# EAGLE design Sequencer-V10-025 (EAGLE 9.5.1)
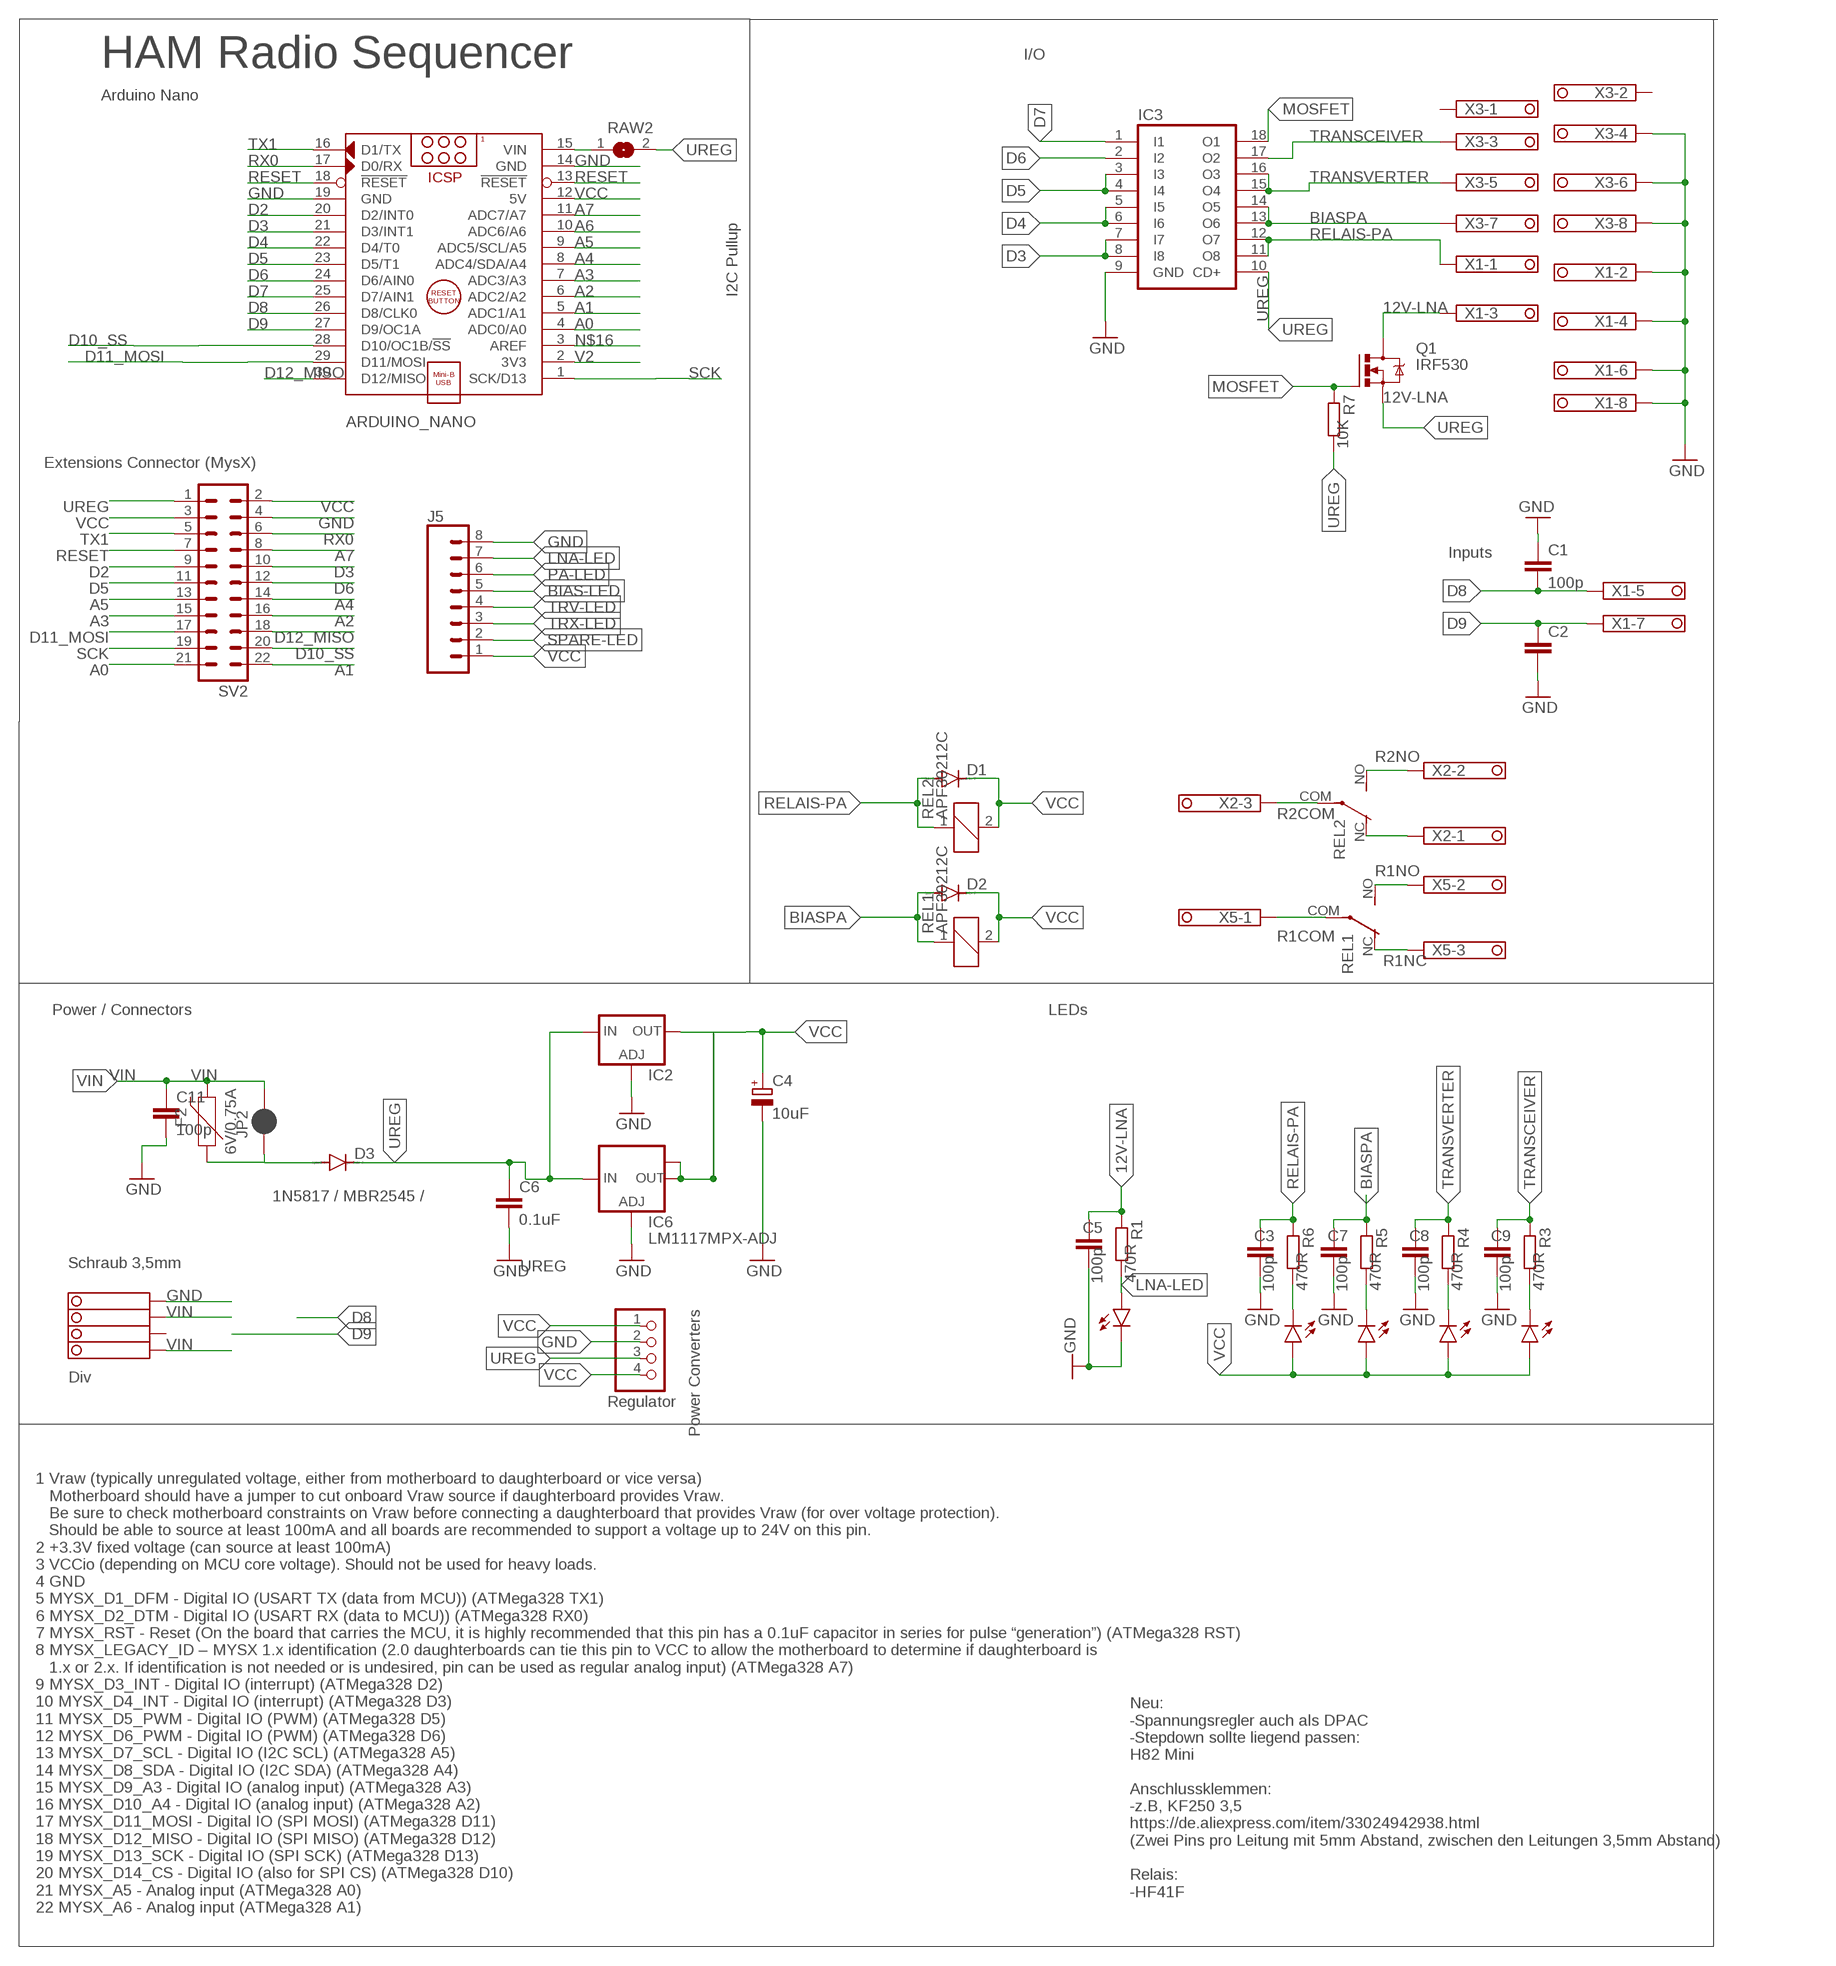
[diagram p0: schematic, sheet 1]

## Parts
ARDUINO_NANO  ARDUINO_NANO_OHNE-BOHR  [ARDUINO_NANO]
C1  100p  C-EU025-025X050  [C025-025X050]
C2  C-EU025-025X050  [C025-025X050]
C3  100p  C-EU025-025X050  [C025-025X050]
C4  10uF  CPOL-EUE3.5-8  [E3,5-8]
C5  100p  C-EU025-025X050  [C025-025X050]
C6  0.1uF  C-EU050-024X044  [C050-024X044]
C7  100p  C-EU025-025X050  [C025-025X050]
C8  100p  C-EU025-025X050  [C025-025X050]
C9  100p  C-EU025-025X050  [C025-025X050]
C11  100p  C-EU025-025X050  [C025-025X050]
D1  DIODE-D-2.5  [D-2.5]
D2  DIODE-D-2.5  [D-2.5]
D3  1N5817 / MBR2545 /  DIODE-D-7.5  [D-7.5]
F2  6V/0.75A  PPTC_THREE-QUARTER-AMP  [1206]
IC2  LD117ADT50TR  [DPACK]
IC3  ULN2803A  [DIL18]
IC6  LM1117MPX-ADJ  [SOT223]
J5  CONN_08LOCK  [1X08_LOCK]
JP2  JUMPER-SMT_2_NC_PASTE_NO-SILK  [SMT-JUMPER_2_NC_PASTE_NO-SILK]
LED-BIAS  LED3MM  [LED3MM]
LED-LNA  LED3MM  [LED3MM]
LED-PA  LED3MM  [LED3MM]
LED-TRV  LED3MM  [LED3MM]
LED-TRX  LED3MM  [LED3MM]
Q1  IRF530  [TO220BV]
R1  470R  R-EU_0207/7  [0207/7]
R3  470R  R-EU_0207/7  [0207/7]
R4  470R  R-EU_0207/7  [0207/7]
R5  470R  R-EU_0207/7  [0207/7]
R6  470R  R-EU_0207/7  [0207/7]
R7  10K  R-EU_0207/7  [0207/7]
RAW2  SJ  [SJ]
REL1  APF30212C  [APF30212C]
REL2  APF30212C  [APF30212C]
STEPDWN  PINHD-1X04_2.54-S  [1X04-S]
SV2  MA11-2  [MA11-2]
X1  MARTIN8X2-1751303  [1751303]
X2  MARTIN3X2-1751303175L303-3  [1751303-3]
X3  MARTIN8X2-1751303  [1751303]
X4  1751264  [1751264]
X5  MARTIN3X2-1751303175L303-3  [1751303-3]

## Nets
12V-LNA: C5.1 Q1.D R1.1 X1.11
A0 [Signal]: ARDUINO_NANO.4(ADC0/A0) SV2.21
A1 [Signal]: ARDUINO_NANO.5(ADC1/A1) SV2.22
A2 [Signal]: ARDUINO_NANO.6(ADC2/A2) SV2.16
A3 [Signal]: ARDUINO_NANO.7(ADC3/A3) SV2.15
A4 [Signal]: ARDUINO_NANO.8(ADC4/SDA/A4) SV2.14
A5 [Signal]: ARDUINO_NANO.9(ADC5/SCL/A5) SV2.13
A6 [Signal]: ARDUINO_NANO.10(ADC6/A6)
A7 [Signal]: ARDUINO_NANO.11(ADC7/A7) SV2.8
BIAS-LED [Signal]: J5.5 LED-BIAS.K(C) R5.2
BIASPA: C7.1 D2.A IC3.13(O6) IC3.14(O5) R5.1 REL1.1 X3.15
D2 [Signal]: ARDUINO_NANO.20(D2/INT0) SV2.9
D3 [Signal]: ARDUINO_NANO.21(D3/INT1) IC3.7(I7) IC3.8(I8) SV2.10
D4 [Signal]: ARDUINO_NANO.22(D4/T0) IC3.5(I5) IC3.6(I6)
D5 [Signal]: ARDUINO_NANO.23(D5/T1) IC3.3(I3) IC3.4(I4) SV2.11
D6 [Signal]: ARDUINO_NANO.24(D6/AIN0) IC3.2(I2) SV2.12
D7 [Signal]: ARDUINO_NANO.25(D7/AIN1) IC3.1(I1)
D8 [Signal]: ARDUINO_NANO.26(D8/CLK0) C1.2 X1.13
D9 [Signal]: ARDUINO_NANO.27(D9/OC1A) C2.1 X1.15
D10_SS [Signal]: ARDUINO_NANO.28(D10/OC1B/!SS) SV2.20
D11_MOSI [Signal]: ARDUINO_NANO.29(D11/MOSI) SV2.17
D12_MISO [Signal]: ARDUINO_NANO.30(D12/MISO) SV2.18
GND [Power]: ARDUINO_NANO.14(GND) ARDUINO_NANO.19(GND) C1.1 C2.2 C3.2 C4.- C5.2 C6.2 C7.2 C8.2 C9.2 C11.2 IC2.1(ADJ) IC3.9(GND) IC6.1(ADJ) J5.8 LED-LNA.K(C) STEPDWN.2 SV2.4 X1.10 X1.12 X1.14 X1.16 X3.12 X3.14 X3.16 X4.4
LNA-LED [Signal]: J5.7 LED-LNA.A R1.2
MOSFET: IC3.18(O1) Q1.G R7.1
N$1: D3.A F2.1 JP2.1
N$16: ARDUINO_NANO.3(AREF)
PA-LED [Signal]: J5.6 LED-PA.K(C) R6.2
R1COM: REL1.COM(2:P) X5.1
R1NC: REL1.NC(2:O) X5.3
R1NO: REL1.NO(2:S) X5.2
R2COM: REL2.COM(2:P) X2.3
R2NC: REL2.NC(2:O) X2.1
R2NO: REL2.NO(2:S) X2.2
RAW1 [Power]: ARDUINO_NANO.15(VIN) RAW2.1
RELAIS-PA: C3.1 D1.A IC3.11(O8) IC3.12(O7) R6.1 REL2.1 X1.9
RESET [Signal]: ARDUINO_NANO.13(!RESET) ARDUINO_NANO.18(!RESET) SV2.7
RX0 [Signal]: ARDUINO_NANO.17(D0/RX) SV2.6
SCK [Signal]: ARDUINO_NANO.1(SCK/D13) SV2.19
SPARE-LED [Signal]: J5.2
TRANSCEIVER: C9.1 IC3.17(O2) R3.1 X3.11
TRANSVERTER: C8.1 IC3.15(O4) IC3.16(O3) R4.1 X3.13
TRV-LED [Signal]: J5.4 LED-TRV.K(C) R4.2
TRX-LED [Signal]: J5.3 LED-TRX.K(C) R3.2
TX1 [Signal]: ARDUINO_NANO.16(D1/TX) SV2.5
UREG [Power]: C6.1 D3.C IC2.3(IN) IC3.10(CD+) IC6.3(IN) Q1.S R7.2 RAW2.2 STEPDWN.3 SV2.1
V2 [Power]: ARDUINO_NANO.2(3V3)
VCC [Power]: ARDUINO_NANO.12(5V) C4.+ D1.C D2.C IC2.4(OUT) IC6.2(OUT) IC6.TAB(OUT1) J5.1 LED-BIAS.A LED-PA.A LED-TRV.A LED-TRX.A REL1.2 REL2.2 STEPDWN.1 STEPDWN.4 SV2.2 SV2.3
VIN [Power]: C11.1 F2.2 JP2.2 X4.1 X4.3
Unconnected: X3.9 X3.10 X4.2

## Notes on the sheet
- I/O
- HAM Radio Sequencer
- Arduino Nano
- I2C Pullup
- Extensions Connector (MysX)
- Inputs
- Power / Connectors | LEDs
- Schraub 3,5mm
- Power Converters
- Div
- Regulator
- Neu:
  -Spannungsregler auch als DPAC
  -Stepdown sollte liegend passen:  
  H82 Mini
  
  Anschlussklemmen:
  -z.B, KF250 3,5 
  https://de.aliexpress.com/item/33024942938.html
  (Zwei Pins pro Leitung mit 5mm Abstand, zwischen den Leitungen 3,5mm Abstand)
  
  Relais:
  -HF41F
- 1 Vraw (typically unregulated voltage, either from motherboard to daughterboard or vice versa)
     Motherboard should have a jumper to cut onboard Vraw source if daughterboard provides Vraw. 
     Be sure to check motherboard constraints on Vraw before connecting a daughterboard that provides Vraw (for over voltage protection). 
     Should be able to source at least 100mA and all boards are recommended to support a voltage up to 24V on this pin.
  2 +3.3V fixed voltage (can source at least 100mA)
  3 VCCio (depending on MCU core voltage). Should not be used for heavy loads.
  4 GND
  5 MYSX_D1_DFM - Digital IO (USART TX (data from MCU)) (ATMega328 TX1)
  6 MYSX_D2_DTM - Digital IO (USART RX (data to MCU)) (ATMega328 RX0)
  7 MYSX_RST - Reset (On the board that carries the MCU, it is highly recommended that this pin has a 0.1uF capacitor in series for pulse “generation”) (ATMega328 RST)
  8 MYSX_LEGACY_ID – MYSX 1.x identification (2.0 daughterboards can tie this pin to VCC to allow the motherboard to determine if daughterboard is 
     1.x or 2.x. If identification is not needed or is undesired, pin can be used as regular analog input) (ATMega328 A7)
  9 MYSX_D3_INT - Digital IO (interrupt) (ATMega328 D2)
  10 MYSX_D4_INT - Digital IO (interrupt) (ATMega328 D3)
  11 MYSX_D5_PWM - Digital IO (PWM) (ATMega328 D5)
  12 MYSX_D6_PWM - Digital IO (PWM) (ATMega328 D6)
  13 MYSX_D7_SCL - Digital IO (I2C SCL) (ATMega328 A5)
  14 MYSX_D8_SDA - Digital IO (I2C SDA) (ATMega328 A4)
  15 MYSX_D9_A3 - Digital IO (analog input) (ATMega328 A3)
  16 MYSX_D10_A4 - Digital IO (analog input) (ATMega328 A2)
  17 MYSX_D11_MOSI - Digital IO (SPI MOSI) (ATMega328 D11)
  18 MYSX_D12_MISO - Digital IO (SPI MISO) (ATMega328 D12)
  19 MYSX_D13_SCK - Digital IO (SPI SCK) (ATMega328 D13)
  20 MYSX_D14_CS - Digital IO (also for SPI CS) (ATMega328 D10)
  21 MYSX_A5 - Analog input (ATMega328 A0)
  22 MYSX_A6 - Analog input (ATMega328 A1)

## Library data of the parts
ARDUINO_NANO = ArduinoNanoV30:ARDUINO_NANO_OHNE-BOHR: Arduino Nano V3.0 Module Overview: The Arduino Nano is a small, complete, and breadboard-friendly board based on the ATmega328 (Arduino Nano 3.x) or ATmega168 (Arduino Nano 2.x). It has more or less the same functionality of the Arduino Duemilanove, but in a different package. It lacks only a DC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
C1-C3 C5-C9 C11 = rcl:C-EU: CAPACITOR, European symbol; SPICEPREFIX: C
C4 = rcl:CPOL-EU: POLARIZED CAPACITOR, European symbol; SPICEPREFIX: C
D1-D3 = diode:DIODE-: DIODE
F2 = SparkFun-Fuses:PPTC: Resettable Fuse PPTC; PROD_ID: RES-11150
IC2 = v-reg:LD117A?*: Low drop fixed and adjustable positive voltage regulators 1 A Source: http://www.st.com/stonline/products/literature/ds/7194/ld1117axx.pdf
IC3 = uln-udn:ULN2803A: DRIVER ARRAY
IC6 = lm1117:LM1117MPX-ADJ
J5 = SparkFun-Connectors:CONN_08: Multi connection point. Often used as Generic Header-pin footprint for 0.1 inch spaced/style header connections On any of the 0.1 inch spaced packages, you can populate with these: Break Away Headers - Straight (PRT-00116) Break Away Male Headers - Right Angle (PRT-00553) Female Headers (PRT-00115)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
JP2 = SparkFun-Jumpers:JUMPER-SMT_2_NC_PASTE: Normally closed solder jumper
LED-BIAS LED-LNA LED-PA LED-TRV LED-TRX = led:LED: LED
Q1 = transistor-power:IRF530: HEXFET Power MOSFET
R1 R3-R7 = rcl:R-EU_: RESISTOR, European symbol; SPICEPREFIX: R
RAW2 = jumper:SJ: SMD solder JUMPER
REL1 REL2 = relay:APF30212C: Compliant with European standards 1a/1c 6A Slim power relays Source: Data sheet; OC_FARNELL: unknown
STEPDWN = pinhead-2:PINHD-1X04: PIN HEADER
SV2 = con-Pinheader:MA11-2: PIN HEADER; OC_FARNELL: unknown; OC_NEWARK: unknown
X1 X3 = con-phoenix-350-Martin:MARTIN8X2-1751303: MKDS 1/ 8-3,5 Printklemme Nennstrom: 10 A Bemessungsspannung: 160 V Raster: 3,5 mm Polzahl: 8 Montageart: Löten Anschlussart: Schraubanschluss Anschlussrichtung vom Leiter zur Platine: 0° Source: http://eshop.phoenixcontact.com .. .pdf; OC_FARNELL: unknown; OC_NEWARK: unknown
X2 X5 = con-phoenix-350-Martin:MARTIN3X2-1751303: MKDS 1/ 8-3,5 Printklemme Nennstrom: 10 A Bemessungsspannung: 160 V Raster: 3,5 mm Polzahl: 8 Montageart: Löten Anschlussart: Schraubanschluss Anschlussrichtung vom Leiter zur Platine: 0° Source: http://eshop.phoenixcontact.com .. .pdf
X4 = con-phoenix-350:1751264: MKDS 1/ 4-3,5 Printklemme Nennstrom: 10 A Bemessungsspannung: 160 V Raster: 3,5 mm Polzahl: 4 Montageart: Löten Anschlussart: Schraubanschluss Anschlussrichtung vom Leiter zur Platine: 0° Source: http://eshop.phoenixcontact.com .. 1751264.pdf; MPN: 1751264; OC_FARNELL: unknown; OC_NEWARK: 10R0934

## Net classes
0 default: width 1.219 mm
1 Power: width 0.762 mm
2 Signal: width 0.305 mm

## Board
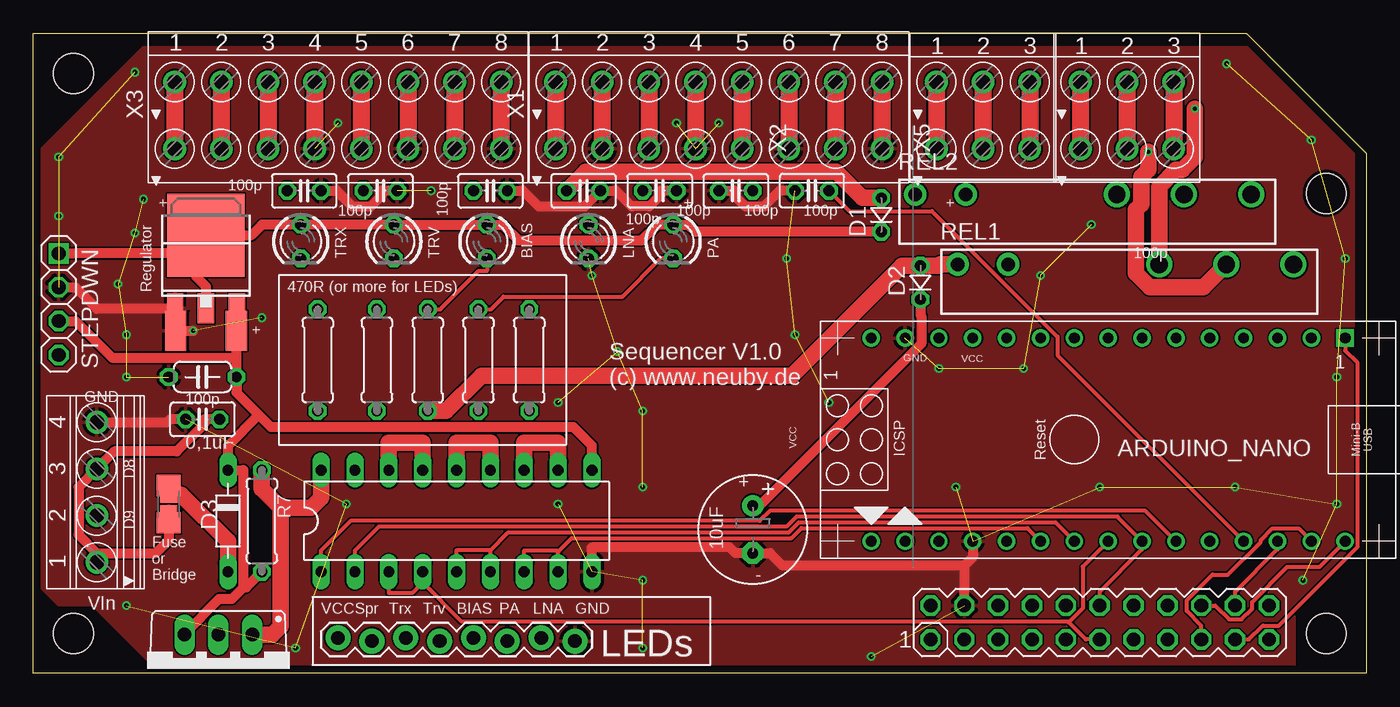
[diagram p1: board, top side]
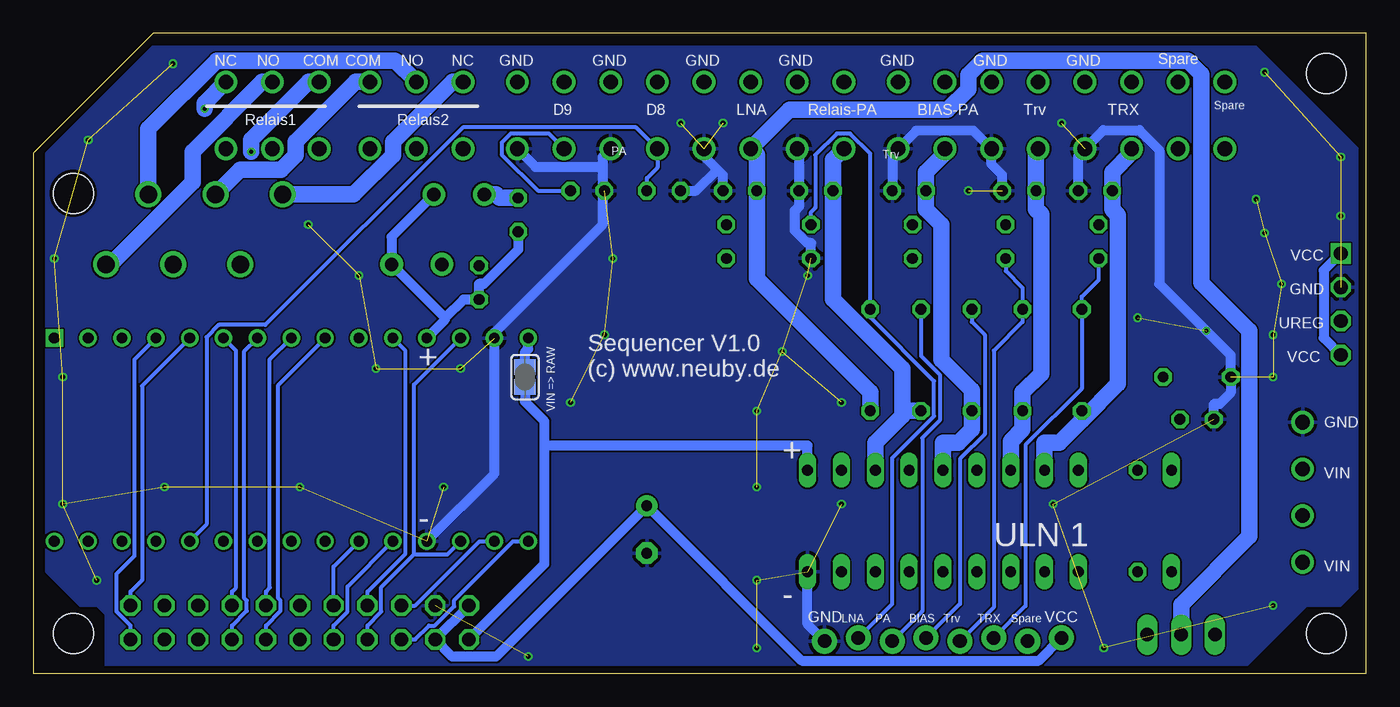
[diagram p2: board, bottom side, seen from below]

Size 100 x 48 mm. Coordinates in mm from the lower left corner, seen from the top.
Outline: 100,0 0,0 0,48 91,48 100,39 100,0
Copper layers (1*16): Top 0.035mm / dielectric 1.5mm / Bottom 0.035mm
Design rules "dirt_cheap_dirty_boards.v1": minimum track width 5mil, minimum drill 12mil, track to track 5mil, track to pad 5mil, pad to pad 5mil, via to via 5mil, smd to smd 0mil, copper to edge 10mil, drill to drill 10mil, minimum pad ring 10mil, minimum via ring 6mil, stop-mask expansion 2mil, vias tented up to drill 25mil, thermal gap 10mil
Holes 3 mm at 3,45 97,36 97,3 3,3

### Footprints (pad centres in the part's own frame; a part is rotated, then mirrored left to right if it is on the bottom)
ARDUINO_NANO = drill 0.8 square: 1 -20.32,-7.62 | drill 0.8: 2 -17.78,-7.62; 3 -15.24,-7.62; 4 -12.7,-7.62; 5 -10.16,-7.62; 6 -7.62,-7.62; 7 -5.08,-7.62; 8 -2.54,-7.62; 9 0,-7.62; 10 2.54,-7.62; 11 5.08,-7.62; 12 7.62,-7.62; 13 10.16,-7.62; 14 12.7,-7.62; 15 15.24,-7.62; 16 15.24,7.62; 17 12.7,7.62; 18 10.16,7.62; 19 7.62,7.62; 20 5.08,7.62; 21 2.54,7.62; 22 0,7.62; 23 -2.54,7.62; 24 -5.08,7.62; 25 -7.62,7.62; 26 -10.16,7.62; 27 -12.7,7.62; 28 -15.24,7.62; 29 -17.78,7.62; 30 -20.32,7.62
C025-025X050 = drill 0.813 octagon: 1 -1.27,0; 2 1.27,0
E3,5-8 = drill 0.813 pad 1.6: + -1.778,0 | drill 0.813 pad 1.6 octagon: - 1.778,0
C050-024X044 = drill 0.813 octagon: 1 -2.54,0; 2 2.54,0
D-2.5 = drill 0.813 octagon: A 1.27,0; C -1.27,0
D-7.5 = drill 0.813 long: A 3.81,0; C -3.81,0
1206 = smd 1.6 x 1.8: 1 -1.4,0; 2 1.4,0
DPACK = smd 1.6 x 3: 1 -2.28,-4.8; 3 2.28,-4.8 | smd 5.8 x 6.2: 4 0,2.38
DIL18 = drill 0.813 long: 1 -10.16,-3.81; 2 -7.62,-3.81; 3 -5.08,-3.81; 4 -2.54,-3.81; 5 0,-3.81; 6 2.54,-3.81; 7 5.08,-3.81; 8 7.62,-3.81; 9 10.16,-3.81; 10 10.16,3.81; 11 7.62,3.81; 12 5.08,3.81; 13 2.54,3.81; 14 0,3.81; 15 -2.54,3.81; 16 -5.08,3.81; 17 -7.62,3.81; 18 -10.16,3.81
SOT223 = smd 1.219 x 2.235: 1 -2.311,-3.099; 2 0,-3.099; 3 2.311,-3.099 | smd 3.6 x 2.2: TAB 0,3.099
1X08_LOCK = drill 1.016 pad 1.88: 1 0,0.127; 2 2.54,-0.127; 3 5.08,0.127; 4 7.62,-0.127; 5 10.16,0.127; 6 12.7,-0.127; 7 15.24,0.127; 8 17.78,-0.127
SMT-JUMPER_2_NC_PASTE_NO-SILK = smd 0.635 x 1.27: 1 -0.406,0; 2 0.406,0
LED3MM = drill 0.813 octagon: A -1.27,0; K 1.27,0
TO220BV = drill 1.016 long: D 0,-2.54; G -2.54,-2.54; S 2.54,-2.54
0207/7 = drill 0.813 octagon: 1 -3.81,0; 2 3.81,0
SJ = smd 1.168 x 1.6: 1 -0.762,0; 2 0.762,0
APF30212C = drill 1 pad 1.7: 1 -12.6,0; 2 -8.82,0 | drill 1.3 pad 1.9: COM 7.56,0; NC 2.52,0; NO 12.6,0
1X04-S = drill 1.016 square: 1 -3.81,0 | drill 1.016 octagon: 2 -1.27,0; 3 1.27,0; 4 3.81,0
MA11-2 = drill 1.016 octagon: 1 -12.7,-1.27; 2 -12.7,1.27; 3 -10.16,-1.27; 4 -10.16,1.27; 5 -7.62,-1.27; 6 -7.62,1.27; 7 -5.08,-1.27; 8 -5.08,1.27; 9 -2.54,-1.27; 10 -2.54,1.27; 11 0,-1.27; 12 0,1.27; 13 2.54,-1.27; 14 2.54,1.27; 15 5.08,-1.27; 16 5.08,1.27; 17 7.62,-1.27; 18 7.62,1.27; 19 10.16,-1.27; 20 10.16,1.27; 21 12.7,-1.27; 22 12.7,1.27
1751303 = drill 1.1 pad 1.7: 1 -12.25,-0.1; 2 -8.75,-0.1; 3 -5.25,-0.1; 4 -1.75,-0.1; 5 1.75,-0.1; 6 5.25,-0.1; 7 8.75,-0.1; 8 12.25,-0.1; 9 -12.25,-5.1; 10 -8.75,-5.1; 11 -5.25,-5.1; 12 -1.75,-5.1; 13 1.75,-5.1; 14 5.25,-5.1; 15 8.75,-5.1; 16 12.25,-5.1
1751303-3 = drill 1.1 pad 1.7: 1 -3.36,2.44; 2 0.14,2.44; 3 3.64,2.44; 4 -3.36,-2.56; 5 0.14,-2.56; 6 3.64,-2.56
1751264 = drill 1.1 pad 1.7: 1 -5.25,-0.1; 2 -1.75,-0.1; 3 1.75,-0.1; 4 5.25,-0.1

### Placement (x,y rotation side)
ARDUINO_NANO  78.11,17.52 180 top
C1  52.7,36.2 0 top
C2  58.42,36.2 180 top
C3  41.27,36.2 0 top
C4  53.98,10.79 270 top
C5  46.99,36.2 0 top
C6  12.7,22.23 180 top
C7  34.29,36.2 0 top
C8  26.04,36.2 0 top
C9  20.32,36.2 0 top
C11  12.7,19.05 180 top
D1  63.62,34.38 90 top
D2  66.56,29.3 90 top
D3  14.61,11.43 270 top
F2  10.16,12.7 270 top
IC2  12.96,30.48 0 top
IC3  31.75,11.43 0 top
IC6  12.96,30.48 0 top
J5  22.86,2.54 0 top
JP2  10.16,12.7 270 top
LED-BIAS  34.03,32.38 270 top
LED-LNA  41.66,32.38 270 top
LED-PA  48.01,32.38 270 top
LED-TRV  27.05,32.38 270 top
LED-TRX  20.07,32.38 270 top
Q1  13.88,0.36 180 top
R1  37.21,23.5 90 top
R3  21.34,23.5 90 top
R4  25.78,23.5 90 top
R5  29.59,23.5 90 top
R6  33.4,23.5 90 top
R7  17.14,11.43 270 top
RAW2  63.12,22.23 270 bottom
REL1  81.94,30.68 0 top
REL2  78.77,35.91 0 top
STEPDWN  1.91,27.68 270 top
SV2  80.01,3.81 0 top
X1  51.44,44.45 0 top
X2  71.12,41.91 0 top
X3  22.86,44.45 0 top
X4  4.67,13.59 90 top
X5  81.92,41.91 0 top

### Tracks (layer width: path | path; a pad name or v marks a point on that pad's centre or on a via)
12V-LNA
  Bottom 1.219: Q1.D 13.88,5.16 8.76,10.29 8.76,25.68 12.36,29.28 12.36,44.93 13.38,45.95 28.79,45.95 29.86,44.88 29.86,43.81 31.41,42.26 43.27,42.26 X1.11 45.72,38.88 C5.1 45.72,29.59 37.21,21.08 R1.1
A0
  Bottom 0.305: SV2.21 92.71,3.58 93.75,4.62 93.75,7.47 92.41,8.81 92.41,23.54 ARDUINO_NANO.4
A1
  Bottom 0.305: ARDUINO_NANO.5 91.85,21.56 91.85,6.99 92.71,6.12 SV2.22
A2
  Bottom 0.305: SV2.16 85.09,6.12 84.78,6.43 84.78,24.2 ARDUINO_NANO.6
A3
  Bottom 0.305: SV2.15 85.09,3.58 83.99,4.68 83.99,5.46 84.17,5.63 84.17,24.16 ARDUINO_NANO.7
A4
  Bottom 0.305: SV2.14 82.55,6.12 82.25,6.42 82.25,23.54 ARDUINO_NANO.8
A5
  Bottom 0.305: SV2.13 82.55,3.58 81.45,4.68 81.45,5.46 81.63,5.63 81.63,21.62 ARDUINO_NANO.9
A7
  Bottom 0.305: SV2.8 74.93,6.12 72.07,8.98 72.07,24.19 ARDUINO_NANO.11
BIAS-LED
  Top 0.305: LED-BIAS.K 34.03,30.18 33.4,30.18 30.53,27.3 R5.2
  Bottom 0.305: R5.2 29.59,26.36 28.62,25.39 28.62,17.94 30.48,16.08 30.48,5.21 J5.5
BIASPA
  Top 1.219: IC3.13 34.29,17.3 31.75,17.3 IC3.14 | R5.1 30.99,19.68 33.62,22.32 56.91,22.32 65.16,30.57 D2.A 67.26,30.57 67.96,30.57 68.06,30.68 REL1.1
  Bottom 1.219: IC3.14 31.75,17.3 30.58,17.3 29.59,18.29 R5.1 29.59,21.25 31.88,23.54 31.88,33.66 33.02,34.8 C7.1 33.02,37.59 31.61,39 X3.15
D2
  Bottom 0.305: SV2.9 77.47,3.58 76.43,4.62 76.43,6.5 ARDUINO_NANO.20
D3
  Top 0.305: 39.37,9.11 40.39,10.13 56.86,10.13 57.62,10.89 74.58,10.89 ARDUINO_NANO.21 | 39.37,9.11 39.26,9.22 36.83,9.22 IC3.7 | IC3.8 39.37,9.11
  Bottom 0.305: SV2.10 77.47,8 ARDUINO_NANO.21
D4
  Top 0.305: 34.29,9.22 35.64,10.57 56.69,10.57 57.44,11.32 76.69,11.32 ARDUINO_NANO.22 | 34.29,9.22 | IC3.6 34.29,9.11 34.29,9.22 | IC3.5 31.75,9.22 34.29,9.22
D5
  Top 0.305: 77.69,3.82 77.62,3.89 32.14,3.89 29.21,6.82 | 77.69,3.82 78.97,2.54 SV2.11 | ARDUINO_NANO.23 78.74,8 78.74,4.87 77.69,3.82 | IC3.3 26.67,6.02 28.41,6.02 29.21,6.82 | IC3.4 29.21,6.82
D6
  Top 0.305: IC3.2 24.13,9.22 25.91,11 56.51,11 57.26,11.76 81.33,11.76 ARDUINO_NANO.24 83.19,9.3 80.01,6.12 SV2.12
D7
  Top 0.305: ARDUINO_NANO.25 83.44,12.19 55.25,12.19 54.49,11.43 23.8,11.43 21.59,9.22 IC3.1
D8
  Bottom 0.305: ARDUINO_NANO.26 87,11.18 87,25.23 86.09,26.13 82.59,26.13 67.77,40.95 54.79,40.95 X1.13 53.19,37.92 53.98,37.13 53.98,36.66 C1.2
D9
  Top 0.305: C2.1 61.23,34.66 67.43,34.66 76.83,25.26 76.83,23.88 ARDUINO_NANO.27
  Bottom 0.305: X1.15 61.31,40.48 64.17,40.48 64.86,39.8 64.86,38.9 62.15,36.2 C2.1
D10_SS
  Top 0.305: SV2.20 90.17,6.12 93.34,9.3 ARDUINO_NANO.28
D11_MOSI
  Top 0.305: SV2.17 87.63,3.58 86.53,4.68 86.53,5.47 88.46,7.39 89.62,7.39 92.08,9.85 92.08,9.97 92.97,10.86 94.93,10.86 ARDUINO_NANO.29
D12_MISO
  Top 0.305: SV2.18 88.67,5.08 89.71,4.04 90.64,4.04 91.44,4.83 91.44,5.34 94.08,7.98 96.5,7.98 ARDUINO_NANO.30
GND  (via drill 0.3 pad 0.61, 0.35)  (41 unrouted)
  Top 0.762: C11.2 10.26,19.05 10.05,18.84 X4.4 | STEPDWN.2 3.17,28.95 4.79,27.34 10.64,27.34 | 10.64,27.34 10.64,27.3 10.64,27.12 10.64,25.75 10.68,25.72 IC2.1 v11.98,25.68 | IC6.1 10.64,27.34 | C7.2 36.73,36.2 37.91,35.01 41.36,35.01 C3.2 43.71,36.2 44.88,35.03 46.22,35.03 47.09,35.9 47.09,36.2 C5.2 | 69.85,8.09 56.21,8.09 55.28,9.02 C4.- 52.67,9.02 52.23,9.45 41.91,9.45 IC3.9 | ARDUINO_NANO.19 70.48,8.72 69.85,8.09 | 69.85,8.09 69.85,6.35 SV2.4 | C8.2 26.14,36.2 26.14,35.83 25.33,35.03 23.93,35.03 22.76,36.2 C9.2 | C1.1 52.6,36.2 52.6,35.83 53.44,34.99 54.78,34.99 55.98,36.2 C2.2
  Bottom 0.762: 57.26,36.2 57.26,33.7 65.41,25.55 ARDUINO_NANO.14 65.41,14.98 ARDUINO_NANO.19 | 57.26,37.99 57.26,38.77 X1.14 | 57.26,36.2 57.26,37.99 | X1.16 62.32,37.99 57.26,37.99 | C2.2 57.26,36.2 | C11.2 11.43,20.22 11,20.22 10.16,21.06 C6.2 10.16,23.86 v11.98,25.68 15.52,29.22 15.52,39.24 17.02,40.73 19.73,40.73 X3.12 21.59,38.87 C9.2 | 48.68,37.78 48.26,37.36 C5.2 | X1.12 49.69,38.79 48.68,37.78 | 48.68,37.78 50.27,36.2 C1.1 | C8.2 27.3,37.36 28.11,38.17 X3.14 29.47,40.71 33.75,40.71 X3.16 35.56,38.9 C7.2 | LED-LNA.K 41.66,32.28 41.95,32.28 42.86,33.2 42.86,34.71 42.55,35.03 C3.2 42.55,39.21 X1.10 | J5.8 41.91,3.68 IC3.9
  other vias: 1.91,38.73 7.62,45.09 7.62,33.02 6.35,29.21 6.99,25.4 6.99,22.23 6.99,5.08 19.68,1.91 23.5,12.7 17.14,26.67 29.84,36.2 41.91,29.84 43.81,24.13 39.37,20.32 59.69,20.32 39.37,12.7 45.72,1.91 45.72,6.99 45.72,13.97 45.72,19.68 56.52,31.11 57.15,25.4 62.87,1.27 69.22,13.97 67.94,22.86 75.56,29.84 79.38,33.66 89.53,45.72 95.89,40.01 98.42,31.11 97.79,22.23 97.79,12.7 90.17,13.97 80.01,13.97 74.3,22.86 95.25,6.99 1.91,34.29 8.26,35.56 22.86,41.27 48.26,41.27 51.44,41.27
  pour Top: 0.64,6.35 0.64,39.37 8.26,46.99 91.08,46.99 99.06,39.01 99.06,7.62 96.52,5.08 95.25,5.08 94.61,4.45 94.61,0.64 8.89,0.64 4.45,5.08 1.91,5.08
  pour Bottom: 8.89,0.64 4.45,5.08 1.91,5.08 0.64,6.35 0.64,39.37 8.26,46.99 91.08,46.99 99.06,39.01 99.06,7.62 96.52,5.08 95.25,5.08 94.61,4.45 94.61,0.64
LNA-LED
  Bottom 0.305: J5.7 35.56,5.21 35.56,16.15 32.43,19.29 32.43,21.91 37.21,26.69 R1.2 37.21,38.97 38.72,40.48 39.72,40.48 41.32,38.88 41.32,34.93 41.66,34.59 LED-LNA.A
MOSFET
  Top 1.219: 18.56,12.43 17.14,13.84 R7.1 | 18.56,12.43 18.56,3.54 17.92,2.9 Q1.G | 18.56,12.43 20.84,12.43 21.59,13.18 IC3.18
N$1
  Top 0.635: 10.16,13.4 JP2.1
  Top 1.219: D3.A 14.61,9.89 11.1,13.4 10.16,13.4 F2.1
PA-LED
  Top 0.305: LED-PA.K 47.06,31.11 44.2,28.25 35.28,28.25 34.34,27.3 R6.2
  Bottom 0.305: R6.2 33.4,23.8 31.99,22.39 31.99,18.98 33.31,17.66 33.31,4.67 J5.6
R1COM  (via drill 0.3 pad 0.61)
  Top 1.219: v83.64,39.11 83.64,37.76 83.12,37.24 83.12,35.16 82.73,34.77 82.73,29.99 83.77,28.95 87.78,28.95 REL1.COM
  Bottom 1.219: X5.1 79.33,44.35 83.64,40.03 v83.64,39.11
R1NC  (via drill 0.3 pad 0.61)
  Top 1.219: v87.14,42.36 87.14,38.69 86.22,37.76 85.72,37.76 84.47,36.51 REL1.NC
  Bottom 1.219: X5.3 87.14,42.76 v87.14,42.36
R1NO
  Bottom 1.219: REL1.NO 94.18,30.68 88.04,36.82 88.04,39.12 82.81,44.35 X5.2
R2COM
  Bottom 1.219: X2.3 75.83,44.35 80.31,39.88 80.31,38.85 81.39,37.76 84.48,37.76 REL2.COM
R2NC
  Bottom 1.219: X2.1 68.55,44.35 73.01,39.89 73.01,38.86 75.95,35.91 REL2.NC
R2NO
  Bottom 1.219: REL2.NO 91.37,40.83 86.26,45.94 72.85,45.94 X2.2
RAW1
  Bottom 0.762: RAW2.1 63.12,24.08 62.87,24.33 ARDUINO_NANO.15
RELAIS-PA
  Top 1.219: D1.A 62.22,35.66 60.27,37.61 41.42,37.61 C3.1 | IC3.11 39.37,17.3 36.83,17.3 IC3.12
  Bottom 1.219: 34.8,19.68 34.8,22.85 40.01,28.05 40.01,34.8 C3.1 40.01,38.53 X1.9 | D1.A 65.02,35.66 65.28,35.91 REL2.1 | R6.1 34.8,19.68 | 34.8,19.68 34.8,19.33 36.83,17.3 IC3.12
RESET
  Bottom 0.305: 71.44,8.93 68.92,8.93 ARDUINO_NANO.18 | 71.44,8.93 73.89,6.47 73.89,4.62 74.93,3.58 SV2.7 | 71.44,8.93 71.44,21.65 ARDUINO_NANO.13
RX0
  Bottom 0.305: SV2.6 71.35,5.08 66.52,9.9 ARDUINO_NANO.17
SCK
  Top 0.305: ARDUINO_NANO.1 98.42,24.21 99.36,23.28 99.36,9.49 93.44,3.58 92.25,3.58 91.21,2.54 SV2.19
TRANSCEIVER
  Bottom 1.219: IC3.17 24.13,17.3 23.02,17.3 21.34,18.99 | 21.34,18.99 18.62,21.7 18.62,34.37 19.05,34.8 C9.1 19.05,37.59 17.61,39.03 X3.11 | R3.1 21.34,18.99
TRANSVERTER
  Top 1.219: IC3.15 29.21,17.3 26.67,17.3 IC3.16
  Bottom 1.219: X3.13 24.77,39.2 C8.1 24.77,34.8 24.38,34.41 24.38,22.48 25.78,21.08 R4.1 25.78,18.99 25.78,18.29 26.67,17.4 IC3.16
TRV-LED
  Bottom 0.305: J5.4 27.94,4.95 27.94,24.2 25.78,26.36 R4.2 25.78,28.91 27.05,30.18 LED-TRV.K
TRX-LED
  Bottom 0.305: J5.3 25.55,5.06 25.55,17.13 21.34,21.35 R3.2 21.34,28.25 20.07,29.52 LED-TRX.K
TX1
  Bottom 0.305: SV2.5 71.35,2.54 70.31,3.58 69.88,3.58 68.43,5.03 68.43,5.48 64.01,9.9 ARDUINO_NANO.16
UREG
  Top 0.762: Q1.S 11.35,2.99 13.94,5.58 14.91,5.58 15.77,6.45 | 15.77,6.45 15.77,15.24 D3.C 14.61,17.07 16.92,19.38 | 16.92,19.38 15.24,21.06 C6.1 15.24,23.67 15.23,23.67 | 16.92,19.38 17.83,18.47 40.51,18.47 41.91,17.07 IC3.10 | STEPDWN.3 3.17,26.41 5.92,23.67 15.23,23.67 | 15.23,23.67 IC2.3 15.27,25.71 IC6.3 | R7.2 15.97,6.45 15.77,6.45
  Bottom 0.762: 61.65,17.07 61.65,18.9 63.12,20.37 RAW2.2 | SV2.1 61.65,8.2 61.65,17.07 | 61.65,17.07 41.91,17.07 IC3.10
VCC
  Top 0.762: D1.C 49.71,33.12 49.17,33.66 LED-PA.A 46.84,33.66 45.65,32.46 36.39,32.46 35.2,33.66 LED-BIAS.A LED-TRV.A LED-TRX.A 17.16,33.66 16.36,32.86 IC2.4 | C4.+ 54.49,12.57 66.62,24.7 66.62,26.81 66.56,26.87 D2.C | IC6.2 12.96,29.01 12.25,29.71 12.25,31.5 | 12.25,31.5 12.25,32.86 IC2.4 | 12.25,31.5 3.17,31.5 STEPDWN.1 | IC6.TAB IC2.4
  Bottom 0.762: J5.1 24.57,0.96 42.36,0.96 C4.+ 65.29,1.26 68.57,1.26 SV2.3 SV2.2 | STEPDWN.1 3.18,30.22 3.18,25.15 STEPDWN.4 | 69.11,26.66 REL1.2 73.12,32.74 REL2.2 | ARDUINO_NANO.12 69.11,26.52 69.11,26.66 | 69.11,26.66 | 69.11,26.66 67.73,28.04 D2.C 66.56,29.2 66.2,29.2 63.62,31.78 D1.C
VIN
  Top 0.635: JP2.2
  Top 0.762: 4.77,9.02 9.19,9.02 10.16,9.99 F2.2 JP2.2 | 4.77,9.02 3.39,10.4 3.39,13.96 X4.3 6.08,16.64 10.76,16.64 12.8,18.69 12.8,19.05 C11.1 | 4.77,9.02 X4.1

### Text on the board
tPlace: VCC | GND | VCC
tNames: 100p | + | + | + | 100p | 100p | 100p | 100p | 100p | 100p | TRX | TRV | BIAS | LNA | PA | 100p | Regulator | 470R (or more for LEDs) | + | Sequencer V1.0 / (c) www.neuby.de | 100p | GND | 0,1uF | D8 | + | 10uF | D9 | Fuse / or / Bridge | - | VIn | VCC | Spr | Trx | Trv | BIAS | PA | LNA | GND | LEDs
bNames: Spare | GND | GND | GND | GND | GND | GND | GND | NC | NO | COM | COM | NO | NC | TRX | Trv | BIAS-PA | Relais-PA | LNA | D8 | D9 | Spare | Relais2 | Relais1 | Trv | PA | VCC | GND | UREG | VIN => RAW | VCC | + | Sequencer V1.0 / (c) www.neuby.de | GND | + | VIN | - | 1 | ULN | VIN | - | VCC | Spare | TRX | Trv | BIAS | PA | LNA | GND
tValues: Gehäuse: Aluminiumgehäuse "1590". Auch genannt,"Gitarren Effekt Gehäuse" von Hammond / Oder: beliebig mit Einschub für 100mm Platinen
